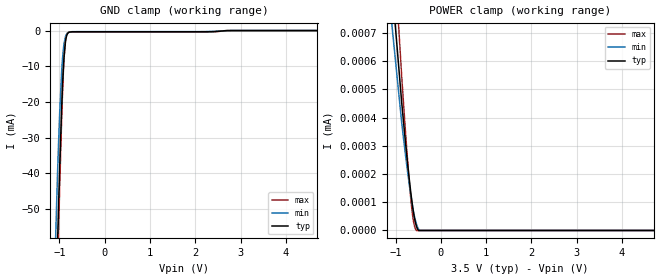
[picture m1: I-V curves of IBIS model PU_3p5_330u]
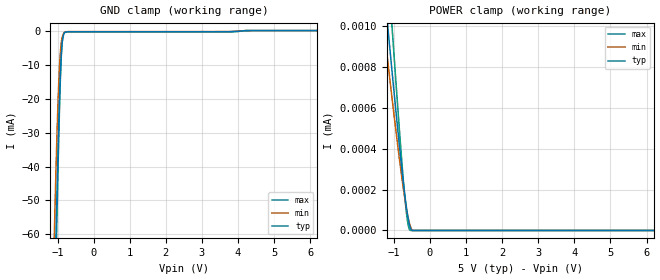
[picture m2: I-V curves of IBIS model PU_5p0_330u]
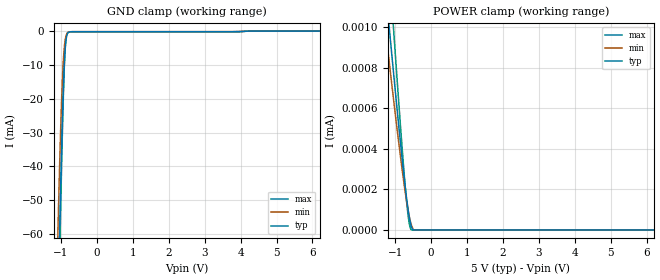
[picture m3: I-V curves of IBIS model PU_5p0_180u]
|Texas Instruments Incorporated
| Marketing part#   Digital Voltage Range   Package-type   #pins
|   TUSB321   4.5V - 5.5V   X2QFN   12
[IBIS Ver]   4.1
[File name]   tusb321.ibs
[File Rev]   1.0
[Date]   06/16/2015
[Source]
| Texas Instruments Incorporated.
| 12500 TI Blvd
| Dallas, TX -75243
[Notes]   Revision History:
| Rev 1.0: 06/08/2015
| - Initial version of the model
| - Model generated from simulations in TISPICE
| - C_comp although listed in numerical order of value are
|   obtained from varying PVT conditions. For PVT conditions for
|   each specific value refer the buffer description under
|   respective [Model]. IBIS model user is responsible for using
|   appropriate C_comp to simulate for Signal Integrity.
| - Warnings regarding combined Non-monotonicity of various models have been
|   reviewd and considered minor and can be ignored.
| - CC1 and CC2 pin have a number of models depending pull-up and pull-down
|   cases (pu_xxx_xxx and pd_xxx respectively). Pull-up model also features
|   dependng on the strength of pull up (pu_xxx_80u, pu_xxx_180u and
|   pu_xxx_330u).
[Disclaimer]
| This model is designed as an aid for customers of Texas Instruments.
| TI and its licensors and suppliers make no warranties, either expressed
| or implied, with respect to this  model, including the warranties of
| merchantability or fitness for a particular purpose. The model is
| provided solely on an "as is" basis. The entire risk as to its quality
| and performance is with the customer.
[Copyright]
 (C) Copyright 2015 Texas Instruments Incorporated.All rights reserved.
|   Device
[Component]  TUSB321
[Manufacturer]   TI
[Package]  |X2QFN   12
|   typ   min   max
R_pkg   0.067   0.027   0.083
L_pkg   0.937nH   0.593nH   1.143nH
C_pkg   0.144pF   0.126pF   0.200pF
[Pin]  signal_name   model_name   R_pin   L_pin   C_pin
1   CC1   CC   NA   NA   NA
2   CC2   CC   NA   NA   NA
3   CURRENT_MODE   NC   NA   NA   NA
4   PORT   ADDR   NA   NA   NA
5   VBUS_DET   NC   NA   NA   NA
6   VCONN_FAULT   INT   NA   NA   NA
7   OUT1   INT   NA   NA   NA
8   OUT2   INT   NA   NA   NA
9   ID   INT   NA   NA   NA
10   GND   GND   NA   NA   NA
11   DIR   INT   NA   NA   NA
12   VDD   POWER   NA   NA   NA
|   Model Selectors
[Model Selector]  CC
PD_5p0  CC1/CC2 buffer at pull-down state at 5.0V VCC.
PU_5p0_80u  CC1/CC2 buffer at 80uA pull-up state at 5.0V VCC.
PU_5p0_180u  CC1/CC2 buffer at 180uA pull-up state at 5.0V VCC.
PU_5p0_330u  CC1/CC2 buffer at 330uA pull-up state at 5.0V VCC.
PU_3p5_330u  CC1/CC2 buffer at 330uA pull-up state at 3.5V VCC.
| Models and submodels in the file (8): PU_3p5_330u (Input), PU_5p0_330u (Input), PU_5p0_180u (Input), PU_5p0_80u (Input), PD_5p0 (Input), INT (Open_drain), DIR (Input), ADDR (Input)
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|   Model
[Model]   PU_3p5_330u
Model_type   Input
Vinl = 1.05
Vinh = 2.45
|   typ   min   max
C_comp   1pF   1pF   1pF
[Voltage Range]   3.5   3.499   3.501
[Temperature Range]   27   105   -40
[Power Clamp Reference]   3.5   3.499   3.501
[GND Clamp Reference]   0   0   0
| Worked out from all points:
|   GND clamp passes 1 mA (typ) near -0.82 V on its own axis
[GND Clamp]
|   Voltage   I(typ)   I(min)   I(max)
-3.5V     -1.465A    -1.389A    -1.519A
-1.127V   -102.9mA   -77.81mA   -113.9mA
-1.043V   -61.2mA    -41.4mA    -69.12mA
-1.032V   -56.28mA   -37.33mA   -63.75mA
-1.022V   -51.45mA   -33.39mA   -58.46mA
-1.012V   -46.73mA   -29.62mA   -53.24mA
-990.5mV  -37.65mA   -22.65mA   -43.12mA
-948.5mV  -21.5mA    -11.48mA   -24.6mA
-906.5mV  -9.498mA   -4.724mA   -10.19mA
-864.5mV  -3.086mA   -1.732mA   -2.644mA
-801.5mV  -618.3uA   -520.7uA   -503.5uA
7V        0A         0A         0A
[POWER Clamp]
|   Voltage   I(typ)   I(min)   I(max)
-3.5V     5.553uA    1.275mA    7.545uA
-3.059V   4.68uA     3.893uA    6.352uA
-864.5mV  452.9nA    381.7nA    545.2nA
-749mV    259.8nA    225.7nA    278.8nA
-707mV    195.2nA    173.8nA    191.3nA
-665mV    135.6nA    125.9nA    113.7nA
-633.5mV  95.61nA    93.52nA    65.69nA
-602mV    61.17nA    64.95nA    30.2nA
-570.5mV  33.83nA    41.04nA    8.968nA
-539mV    14.62nA    22.46nA    0A
-476mV    0A         0A         0A
7V        0A         0A         0A
|   Model
[Model]   PU_5p0_330u
Model_type   Input
Vinl = 1.5
Vinh = 3.5
|   typ   min   max
C_comp   0.475pF   0.451pF   0.489pF
[Voltage Range]   5   4.999   5.001
[Temperature Range]   27   105   -40
[Power Clamp Reference]   5   4.999   5.001
[GND Clamp Reference]   0   0   0
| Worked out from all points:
|   GND clamp passes 1 mA (typ) near -0.82 V on its own axis
[GND Clamp]
|   Voltage   I(typ)   I(min)   I(max)
-5V       -2.345A    -2.242A    -2.422A
-1.085V   -81.6mA    -58.9mA    -91.17mA
-1.04V    -59.78mA   -40.22mA   -67.58mA
-1.025V   -52.82mA   -34.5mA    -59.96mA
-995mV    -39.55mA   -24.07mA   -45.25mA
-965mV    -27.46mA   -15.37mA   -31.53mA
-935mV    -17.1mA    -8.82mA    -19.39mA
-905mV    -9.17mA    -4.562mA   -9.789mA
-890mV    -6.305mA   -3.195mA   -6.319mA
-860mV    -2.706mA   -1.559mA   -2.252mA
-800mV    -603.3uA   -511.5uA   -496uA
10V       0A         0A         0A
[POWER Clamp]
|   Voltage   I(typ)   I(min)   I(max)
-5V       8.523uA    1.593A     11.61uA
-1.91V    2.427uA    87.48uA    3.265uA
-1.25V    1.158uA    959.6nA    1.521uA
-1.145V   960.8nA    797.1nA    1.249uA
-1.04V    766.4nA    637.3nA    979.9nA
-830mV    392.3nA    332.2nA    461.8nA
-695mV    176.2nA    158.2nA    166.7nA
-650mV    114.5nA    108.4nA    88.13nA
-605mV    62.54nA    65.62nA    31.31nA
-530mV    8.341nA    15.64nA    0A
-485mV    0A         0A         0A
10V       0A         0A         0A
|   Model
[Model]   PU_5p0_180u
Model_type   Input
Vinl = 1.5
Vinh = 3.5
|   typ   min   max
C_comp   0.475pF   0.451pF   0.489pF
[Voltage Range]   5   4.999   5.001
[Temperature Range]   27   105   -40
[Power Clamp Reference]   5   4.999   5.001
[GND Clamp Reference]   0   0   0
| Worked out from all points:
|   GND clamp passes 1 mA (typ) near -0.83 V on its own axis
[GND Clamp]
|   Voltage   I(typ)   I(min)   I(max)
-5V       -2.345A    -2.242A    -2.422A
-1.085V   -81.56mA   -58.86mA   -91.13mA
-1.04V    -59.74mA   -40.17mA   -67.54mA
-1.025V   -52.78mA   -34.44mA   -59.92mA
-995mV    -39.5mA    -24mA      -45.2mA
-965mV    -27.4mA    -15.29mA   -31.47mA
-935mV    -17.02mA   -8.721mA   -19.31mA
-905mV    -9.067mA   -4.448mA   -9.683mA
-890mV    -6.19mA    -3.075mA   -6.196mA
-860mV    -2.572mA   -1.431mA   -2.097mA
-800mV    -453.5uA   -376.6uA   -321.8uA
10V       0A         0A         0A
[POWER Clamp]
|   Voltage   I(typ)   I(min)   I(max)
-5V       8.523uA    1.593A     11.61uA
-1.91V    2.427uA    87.48uA    3.265uA
-1.25V    1.158uA    959.6nA    1.521uA
-1.145V   960.8nA    797.1nA    1.249uA
-1.04V    766.4nA    637.3nA    979.9nA
-830mV    392.3nA    332.2nA    461.8nA
-695mV    176.2nA    158.2nA    166.7nA
-650mV    114.5nA    108.4nA    88.13nA
-605mV    62.54nA    65.62nA    31.31nA
-530mV    8.341nA    15.64nA    0A
-485mV    0A         0A         0A
10V       0A         0A         0A
